FUNCTION_BLOCK FB_CylinderTempDiag EXTENDS FB_CylinderTemp
VAR_INPUT
	lrTempMax		AT %I*: LREAL;
	lrTempMin		AT %I*: LREAL;
END_VAR
VAR_OUTPUT
	bError			: BOOL;
	sErrorMsg		: STRING;
END_VAR

// =========================================================
;
// =========================================================

METHOD PUBLIC M_StateMachine : BOOL
VAR_INPUT
	bBasePosReq		: BOOL;
	bWorkPosReq		: BOOL;
END_VAR
// =========================================================

IF NOT bError THEN
	
		// Call the method M_StateMachine of base class FB_Cylinder via 'SUPER^.'
	SUPER^.M_StateMachine(	bBasePosReq := bBasePosReq,
							bWorkPosReq	:= bWorkPosReq );
	
		// Additional diagnosis
	M_StateMachine := M_Diag();
	
END_IF

// =========================================================
END_METHOD

METHOD PUBLIC M_Reset
VAR_INPUT
END_VAR
// =========================================================
	// Reset
	
SUPER^.M_Reset();		// Calling method M_Reset of base class FB_Cylinder via 'SUPER^.'

bError 		:= FALSE;
sErrorMsg 	:= '';

// =========================================================
END_METHOD

METHOD PUBLIC M_Diag : BOOL
VAR_INPUT
END_VAR
// =========================================================
	// Error if temperatur of cylinder is not in accepted interval
	
bError := NOT (lrTempCurrent >= lrTempMin AND lrTempCurrent <= lrTempMax);

IF bError THEN
	
	IF lrTempCurrent > lrTempMax THEN
		sErrorMsg := 'Temperature above maximum';
	ELSE
		sErrorMsg := 'Temperature below minimum';
	END_IF
	
ELSE
	sErrorMsg := '';
END_IF

// =========================================================
	// Return
	
M_Diag := bError;

// =========================================================
END_METHOD

END_FUNCTION_BLOCK
